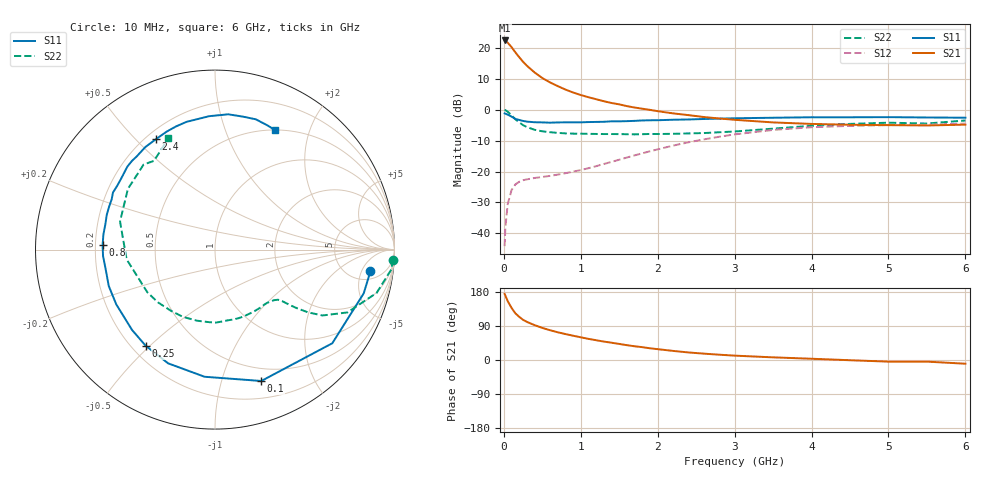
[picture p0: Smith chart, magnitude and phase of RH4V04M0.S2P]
! SIEMENS Small Signal Semiconductors
! BFR106
! Si NPN RF Bipolar Junction Transistor in SOT23
! VCE = 4 V  IC = 4 mA
! Common Emitter S-Parameters:  August  1996
# GHz  S  MA  R  50
!  f  S11  S21  S12  S22
! GHz  MAG  ANG  MAG  ANG  MAG  ANG  MAG  ANG
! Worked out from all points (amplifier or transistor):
!   36 points, 10 MHz to 6 GHz, reference 50 ohm
!   highest |S21| = 22.5 dB at 10 MHz (marker M1)
!   |S21| within 3 dB of that: start of sweep to 125 MHz
!   unconditionally stable (mu >= 1): 669.1 MHz to 1.88 GHz; 4.51 GHz to end of sweep
!   at 250 MHz: K = 0.45, MSG = 19.2 dB, |S12| = -22.8 dB
!   at 1.4 GHz: K = 1.15, MAG = 7.2 dB, |S12| = -16.9 dB
!   at 6 GHz: K = 1.02, MAG = -1.1 dB, |S12| = -4.5 dB
!   S11 on the Smith chart (normalised r, x): 10 MHz: 7, -7; 100 MHz: 0.37, -1.35; 250 MHz: 0.26, -0.49; 800 MHz: 0.23, +0.02; 2.4 GHz: 0.24, +0.57; 6 GHz: 0.50, +1.50
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0.01  0.8742 -8.0  13.27 174.3  0.0062 85.9  0.9939 -3.2
0.02  0.8637 -16.4  13.15 170.1  0.0125 80.5  0.9879 -6.5
0.05  0.8363 -38.6  12.22 155.5  0.0295 70.4  0.9323 -15.0
0.1  0.7761 -70.6  10.36 137.5  0.0501 56.6  0.8162 -25.4
0.15  0.7108 -94.7  8.518 123.1  0.062 46.1  0.7024 -31.5
0.2  0.6854 -112.4  7.108 113.9  0.0684 41.1  0.6252 -34.0
0.25  0.6604 -125.7  5.985 106.0  0.0725 37.1  0.5646 -35.5
0.3  0.6437 -135.8  5.162 100.6  0.0748 36.2  0.5256 -36.4
0.4  0.6291 -151.0  4.024 91.9  0.0788 35.7  0.4748 -37.4
0.5  0.6257 -161.1  3.267 84.7  0.0818 36.9  0.4488 -38.5
0.6  0.6189 -170.0  2.779 78.6  0.0852 39.1  0.4342 -40.4
0.8  0.6267 177.7  2.129 68.5  0.0941 45.5  0.4152 -45.6
1.1  0.6333 162.3  1.598 55.8  0.1134 54.7  0.4082 -55.4
1.3  0.64 154.1  1.377 48.6  0.1327 59.3  0.405 -62.8
1.6  0.6551 143.2  1.147 39.1  0.169 63.0  0.4026 -75.5
2.2  0.6907 124.2  0.876 24.0  0.2633 61.2  0.4087 -104.2
2.4  0.6976 118.2  0.82 19.9  0.2979 58.7  0.4151 -115.5
3.5  0.744 92.5  0.625 7.0  0.4724 37.8  0.4955 -173.7
4.5  0.757 78.1  0.573 -0.6  0.5496 17.5  0.5916 145.1
5  0.7607 72.6  0.565 -4.3  0.5653 9.4  0.6187 130.0
5.5  0.7512 67.1  0.558 -4.3  0.5721 5.3  0.6001 124.5
6  0.7449 63.3  0.575 -9.8  0.5985 -2.6  0.6719 112.8
